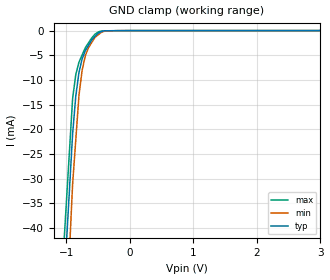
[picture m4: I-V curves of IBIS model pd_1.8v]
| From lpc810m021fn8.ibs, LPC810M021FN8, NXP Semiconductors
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[Model] pd_1.8v
Model_type Input
Vinl = 540.000mV
Vinh = 1.26000V
C_comp 909.000fF 904.000fF 914.000fF
| variable typ   min   max
[Voltage Range] 1.80000V 1.65000V 1.95000V
[POWER Clamp Reference] 1.80000V 1.65000V 1.95000V
[GND Clamp Reference] 0.00000V 0.00000V 0.00000V
[Temperature Range]   25   85   -40
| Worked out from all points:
|   GND clamp passes 1 mA (typ) near -0.53 V on its own axis
[GND Clamp]
-1.8V     -226.1mA   -279.2mA   -207.1mA
-900mV    -20.98mA   -31.13mA   -13.8mA
-850mV    -13.28mA   -22.15mA   -8.911mA
-800mV    -8.483mA   -13.16mA   -6.412mA
-750mV    -5.729mA   -8.059mA   -4.946mA
-700mV    -4.056mA   -5.078mA   -3.479mA
-650mV    -2.988mA   -3.465mA   -2.487mA
-550mV    -1.226mA   -1.411mA   -758.6uA
-500mV    -532.9uA   -883.1uA   -295.9uA
-400mV    -46.91uA   -121.5uA   -71.69uA
-200mV    -8.97uA    -6.932uA   -21.03uA
3.6V      3.469uA    3.969uA    7.534uA
[POWER Clamp]
-1.8V     0A         0A         0A
3.6V      0A         0A         0A
